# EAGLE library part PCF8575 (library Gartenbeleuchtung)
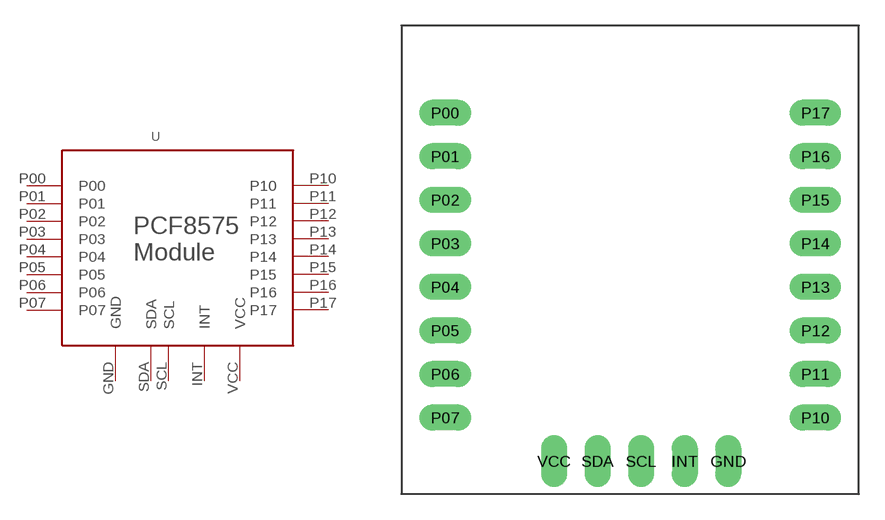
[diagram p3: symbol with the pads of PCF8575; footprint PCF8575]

Designator prefix -

## PCF8575  [PCF8575]
GND  GND  pwr
INT  INT  out
P00  P00
P01  P01
P02  P02
P03  P03
P04  P04
P05  P05
P06  P06
P07  P07
P10  P10
P11  P11
P12  P12
P13  P13
P14  P14
P15  P15
P16  P16
P17  P17
SCL  SCL
SDA  SDA
VCC  VCC  pwr

## Footprint PCF8575 (pad centres in mm)
drill 1 pad 1.422 long: GND 16.51,-2.54; INT 13.97,-2.54; P00 0,17.78; P01 0,15.24; P02 0,12.7; P03 0,10.16; P04 0,7.62; P05 0,5.08; P06 0,2.54; P07 0,0; P10 21.59,0; P11 21.59,2.54; P12 21.59,5.08; P13 21.59,7.62; P14 21.59,10.16; P15 21.59,12.7; P16 21.59,15.24; P17 21.59,17.78; SCL 11.43,-2.54; SDA 8.89,-2.54; VCC 6.35,-2.54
